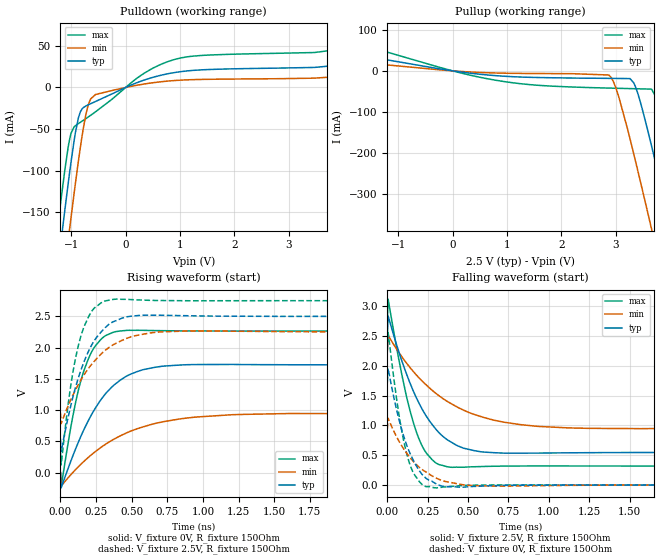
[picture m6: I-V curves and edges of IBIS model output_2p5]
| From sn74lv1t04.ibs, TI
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|   output_2p5 Model
[Model]   output_2p5
Model_type   Output
Polarity   Inverting
Vmeas = 1.25
Vref = 0
Cref = 30pF
Rref = 250
|   typ   min   max
|   (nom PVT)   (fast PVT)   (slow PVT)
C_comp   2.233e-12   2.143e-12   2.287e-12
| Where nom  PVT is Nominal Process, 2.5V, 40C
|   Fast PVT is Strong Process,  2.75V, -40C
|   Slow PVT is Weak Process,   2.25V, 140C
[Voltage Range]   2.5   2.25   2.75
|Junction Temperature
[Temperature Range]   40   140   -40
[Pullup Reference]   2.5   2.25   2.75
[Pulldown Reference]   0   0   0
[Power Clamp Reference]   2.5   2.25   2.75
[GND Clamp Reference]   0   0   0
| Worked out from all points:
|   slope of the pulldown table from 0 to 0.375 V, typ, clamps not added: 38.7 ohm
|   slope of the pullup table from 0 to 0.375 V, typ, clamps not added: 58.5 ohm
|   falling waveform, V_fixture 2.5V, R_fixture 150Ohm: 20-80 % time 214ps typ, 371ps min, 131ps max; typ from 2.5 V to 0.545 V
|   rising waveform, V_fixture 0V, R_fixture 150Ohm: 20-80 % time 264ps typ, 440ps min, 142ps max; typ from 0 V to 1.72 V
|   rising waveform, V_fixture 2.5V, R_fixture 150Ohm: 20-80 % time 178ps typ, 251ps min, 116ps max; typ from 0.545 V to 2.5 V
|   falling waveform, V_fixture 0V, R_fixture 150Ohm: 20-80 % time 127ps typ, 187ps min, 88.4ps max; typ from 1.72 V to 0 V
[Pulldown]
|   Voltage   I(typ)   I(min)   I(max)
-2.5V     -943mA     -1.012A    -893.3mA
-1.353V   -276.1mA   -347.4mA   -224.3mA
-1.193V   -187mA     -257.7mA   -136.5mA
-1.114V   -144.7mA   -214.6mA   -96.63mA
-1.037V   -105.1mA   -173.2mA   -64.17mA
-925mV    -54.38mA   -115.4mA   -45.98mA
-835mV    -29.46mA   -72.52mA   -41.92mA
-688.7mV  -20.81mA   -20.97mA   -35.45mA
-553.7mV  -16.8mA    -8.409mA   -29.22mA
901.8mV   18mA       8.366mA    33.75mA
3.787V    26.08mA    12.64mA    44.74mA
5V        42.93mA    23.14mA    70.79mA
[Pullup]
|   Voltage   I(typ)   I(min)   I(max)
-2.5V     60.3mA     32.97mA    100.9mA
596mV     -9.433mA   -4.39mA    -18.04mA
2.873V    -18.26mA   -10.04mA   -41.81mA
3.006V    -18.42mA   -42.29mA   -42.25mA
3.263V    -18.75mA   -164.5mA   -43.09mA
3.413V    -57.33mA   -245.5mA   -43.58mA
3.66V     -182.5mA   -384.1mA   -44.38mA
3.767V    -241.8mA   -445.1mA   -78.97mA
4.053V    -404.3mA   -609.7mA   -230.3mA
4.252V    -519.3mA   -725.2mA   -343.5mA
4.332V    -565.9mA   -772mA     -389.8mA
5V        -955.6mA   -1.158A    -778.3mA
[Ramp]
R_load = 150
|   typ   min   max
dV/dt_r   1.03297/2.64131e-10   0.563364/4.38309e-10   1.3592/1.42458e-10
dV/dt_f   1.17275/2.1429e-10   0.775145/3.71028e-10   1.45907/1.31233e-10
[Falling Waveform]
V_fixture = 2.5V
V_fixture_min = 2.25V
V_fixture_max = 2.75V
R_fixture = 150Ohm
|   Time   V(typ)   V(min)   V(max)
0s        2.5V       2.25V      2.75V
5ps       2.836V     2.51V      3.117V
115ps     1.89V      2.058V     1.53V
195ps     1.379V     1.801V     780.9mV
275ps     1.025V     1.595V     431.5mV
370ps     761.3mV    1.404V     307mV
475ps     615.7mV    1.251V     298.7mV
665ps     541.5mV    1.084V     315.3mV
1.125ns   540.1mV    957.6mV    319.1mV
3.93ns    545.4mV    958.9mV    318.2mV
[Rising Waveform]
V_fixture = 0V
V_fixture_min = 0V
V_fixture_max = 0V
R_fixture = 150Ohm
|   Time   V(typ)   V(min)   V(max)
0s        402.6pV    6.162nV    602.5pV
5ps       -242.6mV   -212.7mV   -224mV
105ps     372.4mV    46.32mV    1.107V
140ps     563.1mV    127mV      1.443V
190ps     806.7mV    233mV      1.785V
285ps     1.169V     405.4mV    2.133V
390ps     1.426V     553.7mV    2.256V
665ps     1.685V     787mV      2.272V
1.21ns    1.73V      927.2mV    2.264V
5.18ns    1.722V     938.5mV    2.265V
[Rising Waveform]
V_fixture = 2.5V
V_fixture_min = 2.25V
V_fixture_max = 2.75V
R_fixture = 150Ohm
|   Time   V(typ)   V(min)   V(max)
0s        545.4mV    958.1mV    318.2mV
5ps       340.5mV    784.5mV    121.9mV
45ps      791.6mV    1.02V      928.5mV
80ps      1.141V     1.203V     1.502V
145ps     1.647V     1.487V     2.195V
215ps     2.024V     1.722V     2.565V
310ps     2.311V     1.948V     2.744V
460ps     2.489V     2.143V     2.771V
685ps     2.518V     2.248V     2.753V
2.725ns   2.5V       2.249V     2.75V
[Falling Waveform]
V_fixture = 0V
V_fixture_min = 0V
V_fixture_max = 0V
R_fixture = 150Ohm
|   Time   V(typ)   V(min)   V(max)
0s        1.722V     938.9mV    2.265V
5ps       1.954V     1.119V     2.559V
70ps      1.122V     745.9mV    1.215V
95ps      875.2mV    631.6mV    828mV
125ps     632.7mV    515.5mV    475.7mV
165ps     394.9mV    383.4mV    187.2mV
225ps     149mV      242.1mV    -10.5mV
345ps     -22.5mV    70.73mV    -32.3mV
520ps     -25.58mV   -8.422mV   -2.907mV
2.015ns   -52.04uV   817uV      -57.3uV
